(* Logix 5000 AddOnInstructionDefinition export AMCI_SV160E2_Resume; software revision 20.03 *)

ADD_ON_INSTRUCTION AMCI_SV160E2_Resume   (* revision 1.0, vendor AMCI *)
// Revision note:
// 8/2019 Version 0 Initial release of SV160E2 Add On Instructions.
// 3/17/20 Version 1 replaced the generic EDS file with a more complete V1.6 EDS file.
VAR_IN_OUT
   amci_sv160e2_output_data : _000A:SV160E2_9125ACD4:O:0; {required}
END_VAR
VAR
   command_data_block : INT[10];
        [0]   // Command Bits MSW
        [1]   // Command Bits LSW
        [2]   // Upper Target Position
        [3]   // Lower Target Position
        [4]   // Upper Programmed Speed
        [5]   // Lower Programmed Speed
END_VAR

ROUTINE Logic   (* ladder *)
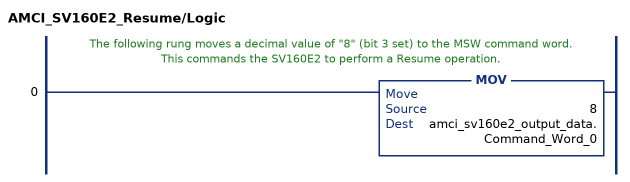
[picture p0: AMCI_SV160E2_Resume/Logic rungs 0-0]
   // The following rung moves a decimal value of "8" (bit 3 set) to the MSW command word.  This commands the SV160E2 to perform a Resume operation.
   0: MOV(8,amci_sv160e2_output_data.Command_Word_0);
END_ROUTINE
END_ADD_ON_INSTRUCTION
